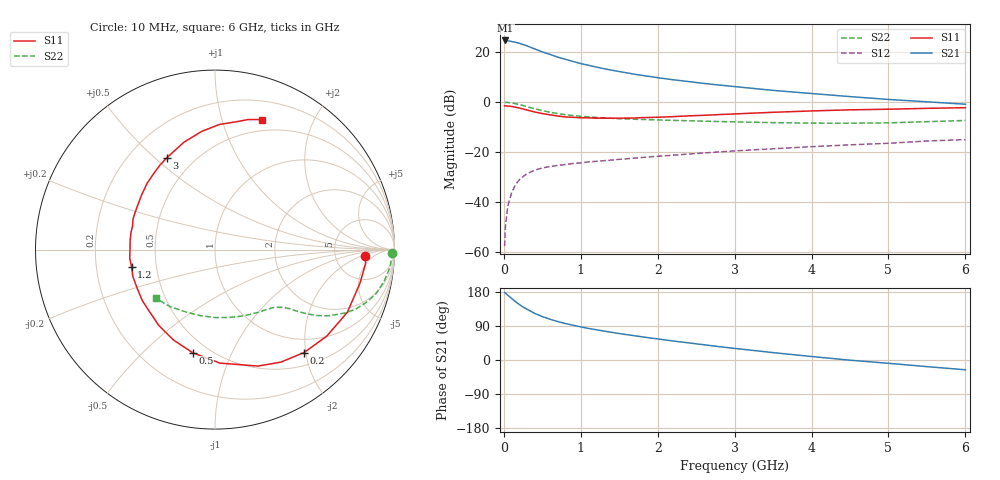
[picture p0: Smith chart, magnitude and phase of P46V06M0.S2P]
! SIEMENS Small Signal Semiconductors
! BFP182
! Si NPN RF Bipolar Junction Transistor in SOT143
! VCE = 6 V  IC = 6 mA
! Common Emitter S-Parameters:  March  1996
# GHz  S  MA  R  50
!  f  S11  S21  S12  S22
! GHz  MAG  ANG  MAG  ANG  MAG  ANG  MAG  ANG
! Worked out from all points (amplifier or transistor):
!   36 points, 10 MHz to 6 GHz, reference 50 ohm
!   highest |S21| = 24.7 dB at 20 MHz (marker M1)
!   |S21| within 3 dB of that: start of sweep to 369.6 MHz
!   unconditionally stable (mu >= 1): 1.531 GHz to 5.561 GHz
!   at 250 MHz: K = 0.23, MSG = 26.4 dB, |S12| = -29.8 dB
!   at 1.4 GHz: K = 0.95, MSG = 18.0 dB, |S12| = -23.2 dB
!   at 6 GHz: K = 0.95, MSG = 7.1 dB, |S12| = -15.0 dB
!   lowest NFmin = 1.25 dB at 450 MHz
!   S11 on the Smith chart (normalised r, x): 10 MHz: 11, -3; 200 MHz: 0.73, -1.97; 500 MHz: 0.41, -0.72; 1.2 GHz: 0.36, -0.09; 3 GHz: 0.36, +0.55; 6 GHz: 0.38, +1.35
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0.01  0.839 -2.5  16.95 178.1  0.0013 94.0  0.9887 -1.0
0.02  0.8423 -5.4  17.1 176.7  0.0031 90.9  0.9828 -2.1
0.05  0.8294 -12.9  16.85 171.1  0.0081 87.0  0.9817 -5.4
0.1  0.8161 -25.3  16.3 162.6  0.0151 76.2  0.9588 -10.6
0.15  0.7874 -37.8  15.77 154.3  0.0217 70.1  0.9296 -15.4
0.2  0.7585 -49.1  15.03 146.7  0.0277 64.7  0.8911 -19.4
0.25  0.7266 -59.6  14.16 139.8  0.0322 60.4  0.8514 -22.9
0.3  0.692 -69.7  13.34 134.0  0.0366 56.3  0.8077 -25.9
0.4  0.633 -87.5  11.6 123.1  0.0432 50.6  0.7338 -30.2
0.5  0.588 -102.2  10.09 114.6  0.0479 45.7  0.6741 -33.0
0.6  0.5542 -114.7  8.993 107.5  0.0511 42.7  0.6255 -34.9
0.7  0.5259 -126.6  7.929 101.5  0.0538 40.8  0.5873 -36.3
0.8  0.5019 -137.0  7.171 96.2  0.056 39.3  0.5584 -37.4
1.1  0.4816 -161.7  5.448 83.3  0.0632 37.0  0.5041 -40.0
1.2  0.4748 -168.4  5.024 79.9  0.065 36.6  0.4917 -40.9
1.7  0.4781 163.8  3.599 64.0  0.0754 36.5  0.4523 -46.1
2.2  0.5099 143.2  2.791 50.2  0.0862 35.7  0.43 -53.1
3  0.5778 117.8  2.039 30.6  0.1049 33.0  0.4004 -67.4
3.5  0.623 106.1  1.711 19.5  0.1159 30.2  0.3866 -78.0
4.5  0.6979 87.9  1.285 -0.5  0.1387 24.7  0.3769 -102.5
5.5  0.7477 75.7  1.011 -17.5  0.1658 19.1  0.4046 -128.2
6  0.7698 70.2  0.904 -25.8  0.1771 14.8  0.427 -140.7
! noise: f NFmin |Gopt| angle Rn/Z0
0.45  1.25  0.25  39  0.3
0.9  1.4  0.25  78  0.23
1.8  1.95  0.21  151  0.2
